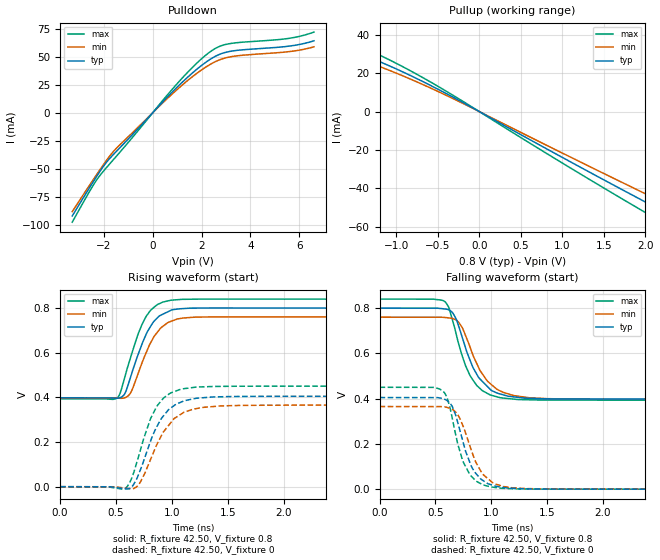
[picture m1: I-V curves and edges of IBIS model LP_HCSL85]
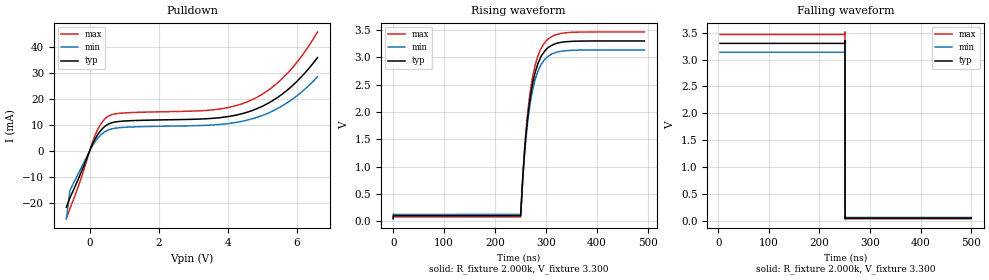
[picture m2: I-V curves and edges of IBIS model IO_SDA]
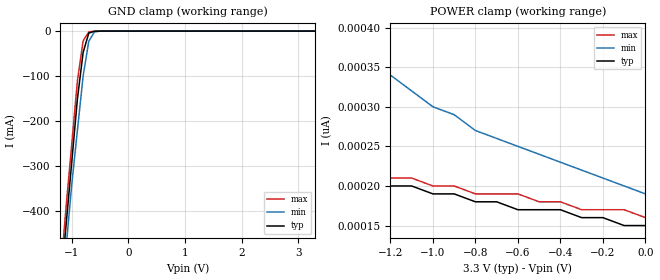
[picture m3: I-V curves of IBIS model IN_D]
| Integrated Devices Technolgy, Inc
[IBIS Ver]   4.1
[File name]   9zxl0651.ibs
[File Rev]   1.1
[Date]   August 12, 2013
|Rev history   1.1
|   Rev 1.1   August 8, 2013  update IO_SDA
|   Rev 1.0   Arpil, 2013  initial revison
[Disclaimer] Integrated Device Technology, Inc. ("IDT") hereby grants the
   user of this ibis model a non-exclusive, nontransferable
   license to use this ibis model under the following terms. the
   user is granted this license only to use the ibis model and is
   not granted rights to sell, copy (except as needed to run the
   ibis model), rent, lease or sub-license the ibis model in
   whole or in part, or in modified form to anyone. the user may
   modify the ibis model to suit its specific applications, but
   rights to derivative works and such modifications shall belong
   to idt. this ibis model is provided on an as is" basis and idt
   makes absolutely no warranty with respect to the information
   contained herein. idt disclaims and customer waives all
   warranties, express and implied, including warranties of
   merchantability and fitness for a particular purpose. the
   entire risk as to quality and performance is with the user
   accordingly, in no event shall idt be liable for any direct or
   indirect damages, whether in contract or tort, including any
   lost profits or other incidental, consequential, exemplary, or
   punitive damages arising out of the use or application of the
   ibis model. further, idt reserves the right to make changes
   without notice to any product herein to improve reliability,
   function, or design. idt does not convey any license under
   patent rights or any other intellectual property rights,
   including those of third parties. idt is not obligated to
   provide maintenance or support for the licensed ibis model.
[Copyright]   Copyright 2012, Integrated Devices Technolgy, Inc. all rights
   reserved
[Component]   9zxl0651
[Manufacturer] Integrated Device Technology, Inc.
[Package]
R_pkg   81.1m   62.2m   100.0m
L_pkg   6.7nH   4.9nH   8.5nH
C_pkg   0.53pF   0.21pF   0.85pF
[Pin] signal_name  model_name
1   VDDA   POWER
2   HIBW_BYPM_LOBW#   IN
3   CKPWRGD_PD#   IN
4   GND   GND
5   VDDR   POWER
6   DIF_IN   IN_DIFF
7   DIF_IN#   IN_DIFF
8   SMBDAT   IO_SDA
9   SMBCLK   IN_D
10   DFB_OUT_NC#   LP_HCSL85
11   DFB_OUT_NC   LP_HCSL85
12   VDD   POWER
13   OE0#   IN
14   DIF_0   LP_HCSL85
15   DIF_0#   LP_HCSL85
16   VDD   POWER
17   DIF_1   LP_HCSL85
18   DIF_1#   LP_HCSL85
19   OE1#   IN
20   VDD   POWER
21   VDD   POWER
22   OE2#   IN
23   DIF_2   LP_HCSL85
24   DIF_2#   LP_HCSL85
25   VDD   POWER
26   DIF_3   LP_HCSL85
27   DIF_3#   LP_HCSL85
28   OE3#   IN
29   VDD   POWER
30   NC   NC
31   VDD   POWER
32   OE4#   IN
33   DIF_4   LP_HCSL85
34   DIF_4#   LP_HCSL85
35   VDD   POWER
36   DIF_5   LP_HCSL85
37   DIF_5#   LP_HCSL85
38   OE5#   IN
39   VDD   POWER
40   NC   NC
[Diff Pin]  inv_pin  vdiff tdelay_typ tdelay_min  tdelay_max
6   7   NA   0   0   0
11   10   NA   0   0   0
14   15   NA   0   0   0
17   18   NA   0   0   0
23   24   NA   0   0   0
26   27   NA   0   0   0
33   34   NA   0   0   0
36   37   NA   0   0   0
| Models and submodels in the file (5): LP_HCSL85 (Output), IO_SDA (I/O_open_drain), IN_D (Input), IN (Input), IN_DIFF (Input)
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|   Model LP_HCSL85   LPRS type output
[Model]   LP_HCSL85
Model_type   Output
Polarity   Non-Inverting
|   typ   min   max
C_comp   2pF   1.5pF   2.5pF
Vmeas = 0.4V
Rref = 42.50
Cref = 0
Vref = 0.4V
|   typ   min   max
[Voltage range]   0.8V   0.76V   0.84V
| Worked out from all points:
|   slope of the pulldown table from 0 to 0.12 V, typ, clamps not added: 41.9 ohm
|   slope of the pullup table from 0 to 0.12 V, typ, clamps not added: 41.3 ohm
|   rising waveform, R_fixture 42.50, V_fixture 0.8: 20-80 % time 189ps typ, 192ps min, 183ps max; typ from 0.398 V to 0.8 V
|   falling waveform, R_fixture 42.50, V_fixture 0.8: 20-80 % time 207ps typ, 219ps min, 185ps max; typ from 0.8 V to 0.398 V
|   rising waveform, R_fixture 42.50, V_fixture 0: 20-80 % time 213ps typ, 230ps min, 191ps max; typ from 0 V to 0.405 V
|   falling waveform, R_fixture 42.50, V_fixture 0: 20-80 % time 162ps typ, 178ps min, 150ps max; typ from 0.405 V to 0 V
[Pulldown]
|Voltage   I (typ)   I (min)   I (max)
|Note, modeling breaks down at 250mA and above.  This is well beyond the functional   |
|operating range of the device.  Should this scenario occur, catastrophic failure and   |
|possible damage to the device and/or board is of higher concern than the I-V curve   |
|behavior.  The IBIS checker will flag currents in excess of 10A with warnings.  Lines   |
|with currents in excess of 0.35 A have been commented out.  The points still remain|
|available to the user if the user desires to use them.   |
-3.3V     -92.31mA   -88.47mA   -97.85mA
-2.391V   -60.06mA   -58.27mA   -63.12mA
-1.987V   -46.86mA   -45.35mA   -51.42mA
-1.583V   -36.66mA   -33.96mA   -41.21mA
942.9mV   21.57mA    19.59mA    24.51mA
1.65V     35.92mA    32.56mA    40.96mA
2.256V    46.26mA    41.84mA    52.83mA
2.66V     51.37mA    46.5mA     58.45mA
3.064V    54.27mA    49.34mA    61.27mA
5.489V    59.14mA    54.26mA    66.08mA
6.095V    61.27mA    56.17mA    68.58mA
6.6V      64.15mA    58.76mA    71.93mA
[Pullup]
|Voltage   I (typ)   I (min)   I (max)
|Note, modeling breaks down at 250mA and above.  This is well beyond the functional   |
|operating range of the device.  Should this scenario occur, catastrophic failure and   |
|possible damage to the device and/or board is of higher concern than the I-V curve   |
|behavior.  The IBIS checker will flag currents in excess of 10A with warnings.  Lines   |
|with currents in excess of 0.35 A have been commented out.  The points still remain|
|available to the user if the user desires to use them.   |
-3.3V     40.69mA    38.06mA    43.93mA
-2.088V   37.36mA    34.26mA    41.15mA
-1.785V   34.77mA    31.57mA    38.86mA
-1.381V   29.13mA    26.28mA    32.9mA
-976.5mV  21.77mA    19.61mA    24.63mA
-471.4mV  11.04mA    9.947mA    12.49mA
1.549V    -36.73mA   -33.33mA   -41.11mA
2.256V    -52.96mA   -48.17mA   -59.04mA
2.357V    -55.24mA   -50.25mA   -61.55mA
2.559V    -59.76mA   -54.39mA   -66.53mA
2.862V    -66.41mA   -60.49mA   -73.81mA
6.6V      -184.6mA   -175mA     -196.4mA
[Ramp]
|   typ   min   max
dV/dt_r   0.242/0.19n   0.218/0.192n   0.269/0.184n
dV/dt_f   0.241/0.207n   0.217/0.219n   0.268/0.184n
R_load =   42.50
[Rising Waveform]
R_fixture = 42.50
V_fixture = 0.8   |Vcc_typ
V_fixture_min = 0.76 |Vcc_min
V_fixture_max = 0.84 |Vcc_max
C_fixture = 0.0p
| Time   typ   min   max
0s        398mV      397.7mV    393.4mV
510ps     396.1mV    396.5mV    397.5mV
570ps     409.9mV    397.2mV    475.6mV
630ps     490.9mV    419.6mV    578.5mV
700ps     595mV      510.2mV    686.6mV
770ps     682.8mV    600.2mV    763.1mV
890ps     765.4mV    704.9mV    820.1mV
990ps     789.6mV    740.1mV    835mV
1.33ns    800.4mV    760.5mV    840.2mV
5ns       800mV      760mV      840mV
[Falling Waveform]
R_fixture = 42.50
V_fixture = 0.8   |Vcc_typ
V_fixture_min = 0.76 |Vcc_min
V_fixture_max = 0.84 |Vcc_max
C_fixture = 0.0p
| Time   typ   min   max
0s        800mV      760mV      840mV
590ps     796.1mV    758.5mV    826.6mV
620ps     792.3mV    756.9mV    803.1mV
690ps     747.7mV    745.5mV    676.5mV
740ps     671.8mV    714.4mV    588.7mV
810ps     570mV      627.7mV    501.8mV
900ps     486.4mV    523.7mV    444.5mV
1.08ns    420.5mV    433.9mV    404.1mV
1.62ns    398.5mV    398.7mV    393.5mV
5ns       398mV      397.7mV    393.4mV
[Rising Waveform]
R_fixture = 42.50
V_fixture = 0
C_fixture = 0.0p
| Time   typ   min   max
0s        610.5nV    -267.7nV   -549.3nV
590ps     -9.934mV   -7.291mV   -4.511mV
650ps     3.92mV     -8.804mV   50.81mV
710ps     65.23mV    14.57mV    149mV
800ps     191.2mV    111mV      292.2mV
860ps     264.1mV    183.3mV    355.3mV
970ps     344.7mV    274mV      413.5mV
1.09ns    380.5mV    327.5mV    437.8mV
1.56ns    404mV      363.6mV    449.8mV
4.97ns    404.9mV    365.3mV    450.2mV
[Falling Waveform]
R_fixture = 42.50
V_fixture = 0
C_fixture = 0.0p
| Time   typ   min   max
0s        404.9mV    365.3mV    450.2mV
570ps     399.3mV    364.5mV    432mV
610ps     389.9mV    360.5mV    395.6mV
650ps     366.5mV    353.1mV    314.5mV
750ps     203.5mV    275.7mV    119mV
850ps     77.09mV    132.5mV    42.68mV
920ps     40.12mV    67.5mV     20.49mV
990ps     20.7mV     38.03mV    10.35mV
1.43ns    591.1uV    980.6uV    267.9uV
5ns       29.58nV    -29.14nV   -8.363uV
|   Model IO_SDA
[Model]   IO_SDA
Model_type   I/O_open_drain
Polarity   Inverting
Vinl = 0.80V
Vinh = 2.10V
|   typ   min   max
C_comp   2pF   1.5pF   2.5pF
Vmeas = 1.65V
Rref = 2000
Cref = 0
Vref = 1.65V
|   typ   min   max
[Voltage range]   3.3V   3.135V   3.465V
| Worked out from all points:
|   slope of the pulldown table from 0 to 0.495 V, typ, clamps not added: 49.7 ohm
|   rising waveform, R_fixture 2.000k, V_fixture 3.300: 20-80 % time 23.1ns typ, 23.1ns min, 23.1ns max; typ from 0.052 V to 3.3 V
|   falling waveform, R_fixture 2.000k, V_fixture 3.300: 20-80 % time 162ps typ, 198ps min, 134ps max; typ from 3.3 V to 0.05 V
[Pulldown]
|Voltage   I (typ)   I (min)   I (max)
|Note, modeling breaks down at 250mA and above.  This is well beyond the functional   |
|operating range of the device.  Should this scenario occur, catastrophic failure and   |
|possible damage to the device and/or board is of higher concern than the I-V curve   |
|behavior.  The IBIS checker will flag currents in excess of 10A with warnings.  Lines   |
|with currents in excess of 0.35 A have been commented out.  The points still remain|
|available to the user if the user desires to use them.   |
|-3.30000e+00   -1.13615e+02   -1.01878e+02   -1.31507e+02
|-3.19898e+00   -1.08858e+02   -9.77507e+01   -1.25809e+02
|-3.09796e+00   -1.04101e+02   -9.36230e+01   -1.20111e+02
|-2.99694e+00   -9.93436e+01   -8.94951e+01   -1.14413e+02
|-2.89592e+00   -9.45864e+01   -8.53672e+01   -1.08715e+02
|-2.79490e+00   -8.98292e+01   -8.12392e+01   -1.03016e+02
|-2.69388e+00   -8.50718e+01   -7.71111e+01   -9.73181e+01
|-2.59286e+00   -8.03144e+01   -7.29830e+01   -9.16198e+01
|-2.49184e+00   -7.55568e+01   -6.88547e+01   -8.59213e+01
|-2.39082e+00   -7.07992e+01   -6.47263e+01   -8.02228e+01
|-2.28980e+00   -6.60415e+01   -6.05979e+01   -7.45242e+01
|-2.18878e+00   -6.12838e+01   -5.64694e+01   -6.88255e+01
|-2.08776e+00   -5.65259e+01   -5.23408e+01   -6.31267e+01
|-1.98673e+00   -5.17680e+01   -4.82121e+01   -5.74279e+01
|-1.88571e+00   -4.70100e+01   -4.40834e+01   -5.17291e+01
|-1.78469e+00   -4.22520e+01   -3.99546e+01   -4.60301e+01
|-1.68367e+00   -3.74939e+01   -3.58257e+01   -4.03312e+01
|-1.58265e+00   -3.27358e+01   -3.16968e+01   -3.46321e+01
|-1.48163e+00   -2.79776e+01   -2.75678e+01   -2.89331e+01
|-1.38061e+00   -2.32194e+01   -2.34389e+01   -2.32340e+01
|-1.27959e+00   -1.84612e+01   -1.93099e+01   -1.75350e+01
|-1.17857e+00   -1.37030e+01   -1.51809e+01   -1.18359e+01
|-1.07755e+00   -8.94493e+00   -1.10520e+01   -6.13695e+00
|-9.76531e-01   -4.18691e+00   -6.92316e+00   -7.42504e-01
|-8.75510e-01   -3.68185e-01   -2.79449e+00   -4.31911e-02
|-7.74490e-01   -3.36743e-02   -2.18476e-01   -3.07793e-02
-673.5mV  -21.72mA   -26.22mA   -25.8mA
-572.4mV  -18.12mA   -15.39mA   -22.28mA
-471.4mV  -15.15mA   -12.43mA   -18.87mA
134.7mV   4.016mA    3.132mA    5.303mA
336.7mV   8.119mA    6.349mA    10.64mA
538.8mV   10.32mA    8.079mA    13.39mA
3.569V    12.55mA    9.995mA    15.82mA
4.58V     14.97mA    11.89mA    18.97mA
5.085V    17.74mA    14.08mA    22.55mA
5.59V     21.99mA    17.44mA    28mA
6.095V    27.99mA    22.19mA    35.67mA
6.6V      35.95mA    28.52mA    45.79mA
[Ramp]
|   typ   min   max
dV/dt_r   1.979/23.114n   1.88/23.072n   2.078/23.067n
dV/dt_f   1.984/0.165n   1.944/0.21n   2.092/0.136n
R_load =   2000
[Rising Waveform]
R_fixture = 2.000k
V_fixture = 3.300
V_fixture_min = 3.135
V_fixture_max = 3.465
C_fixture = 0.000
|  time   V(typ)   V(min)   V(max)
0s        51.51mV    63.56mV    39.94mV
646.4ps   107.5mV    130.1mV    83.55mV
250.3ns   100.6mV    123.6mV    78.58mV
254.1ns   734.4mV    710.5mV    752.5mV
258.3ns   1.308V     1.257V     1.361V
267.3ns   2.137V     2.042V     2.241V
278.7ns   2.72V      2.588V     2.853V
296.4ns   3.1V       2.95V      3.255V
334.3ns   3.281V     3.116V     3.445V
493.4ns   3.3V       3.135V     3.465V
[Falling Waveform]
R_fixture = 2.000k
V_fixture = 3.300
V_fixture_min = 3.135
V_fixture_max = 3.465
C_fixture = 0.000
|  time   V(typ)   V(min)   V(max)
3.422ns   3.3V       3.135V     3.465V
250.3ns   3.325V     3.146V     3.513V
250.4ns   3.348V     3.166V     3.473V
250.4ns   3.332V     3.183V     3.172V
250.5ns   2.923V     3.084V     2.169V
250.6ns   1.482V     2.246V     276.4mV
250.7ns   520.1mV    1.487V     34.55mV
250.8ns   48.19mV    416.2mV    48.09mV
250.9ns   61.39mV    61.07mV    42.66mV
500ns     49.88mV    63.56mV    39.94mV
|   Model IN_D
[Model]   IN_D
Model_type   Input
Polarity   Inverting
Enable   Active-High
Vinl =   1.00V
Vinh =   2.00V
C_comp   3.40pF   2.85pF   3.95pF
[Temperature Range]   27.00   70.00   0.000
[Voltage Range]   3.30V   3.00V   3.60V
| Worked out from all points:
|   GND clamp passes 1 mA (typ) near -0.62 V on its own axis
[GND_clamp]
| voltage   I(typ)   I(min)   I(max)
-3.3V     -3.78A     -3.65A     -3.87A
-1.2V     -570mA     -610mA     -540mA
-1.1V     -430mA     -480mA     -390mA
-1V       -290mA     -340mA     -250mA
-900mV    -150mA     -220mA     -110mA
-800mV    -47.77mA   -100mA     -21.77mA
-700mV    -4.42mA    -22.5mA    -1.71mA
-600mV    -390uA     -1.83mA    -190uA
-500mV    -33.14uA   -140uA     -13.41uA
3.3V      150pA      220pA      150pA
[POWER_clamp]
| voltage   I(typ)   I(min)   I(max)
-3.3V     350pA      1.67nA     300pA
-2.6V     280pA      890pA      270pA
-2.5V     280pA      820pA      260pA
-2.3V     260pA      700pA      260pA
-2.2V     250pA      640pA      250pA
-1.5V     220pA      400pA      220pA
-1.4V     210pA      380pA      220pA
-1V       190pA      300pA      200pA
-800mV    180pA      270pA      190pA
-600mV    170pA      250pA      190pA
-400mV    170pA      230pA      180pA
0V        150pA      190pA      160pA
